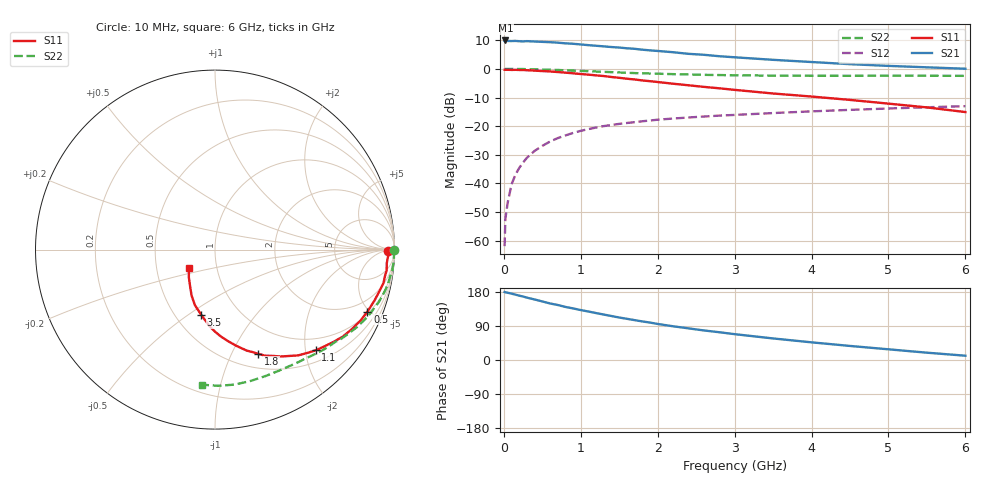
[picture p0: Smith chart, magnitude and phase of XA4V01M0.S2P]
! SIEMENS Discrete & RF Semiconductors
! BFY180
! Si NPN RF Bipolar Junction Transistor in MICRO-X
! VCE = 4 V  IC = 1 mA
! Common Emitter S-Parameters:  May  1997
# GHz  S  MA  R  50
!  f  S11  S21  S12  S22
! GHz  MAG  ANG  MAG  ANG  MAG  ANG  MAG  ANG
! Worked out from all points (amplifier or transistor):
!   36 points, 10 MHz to 6 GHz, reference 50 ohm
!   highest |S21| = 9.9 dB at 20 MHz (marker M1)
!   |S21| within 3 dB of that: start of sweep to 1.726 GHz
!   unconditionally stable (mu >= 1): 3.982 GHz to end of sweep
!   at 250 MHz: K = 0.06, MSG = 21.2 dB, |S12| = -32.7 dB
!   at 1.4 GHz: K = 0.50, MSG = 13.6 dB, |S12| = -19.6 dB
!   at 6 GHz: K = 1.06, MAG = 5.1 dB, |S12| = -13.0 dB
!   S11 on the Smith chart (normalised r, x): 10 MHz: 56, -8; 500 MHz: 1.12, -4.87; 1.1 GHz: 0.73, -2.21; 1.8 GHz: 0.66, -1.27; 3.5 GHz: 0.67, -0.56; 6 GHz: 0.73, -0.15
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0.01  0.9657 -0.3  3.059 179.4  0.0008 73.3  0.9984 -0.2
0.02  0.9643 -0.9  3.141 178.6  0.0024 84.6  0.9999 -0.5
0.05  0.9654 -2.0  3.077 177.5  0.0046 84.1  0.9968 -1.3
0.1  0.96 -4.5  3.065 175.1  0.0096 87.6  0.9979 -2.7
0.15  0.9634 -6.9  3.084 172.5  0.0141 85.5  0.9983 -4.0
0.25  0.957 -11.2  3.025 167.5  0.0232 83.5  0.9947 -6.7
0.3  0.9483 -13.3  3.056 164.6  0.028 81.0  0.9888 -7.9
0.5  0.9169 -22.1  2.968 154.5  0.0452 74.6  0.9767 -13.0
0.6  0.9022 -26.0  2.929 149.2  0.0538 71.7  0.9674 -15.5
0.7  0.8817 -30.2  2.876 145.2  0.0617 68.7  0.9578 -17.9
0.8  0.861 -34.3  2.797 140.1  0.0688 66.4  0.9451 -20.2
1.1  0.7938 -45.0  2.6 127.9  0.0888 58.8  0.9118 -26.6
1.5  0.6993 -58.4  2.361 112.1  0.1096 50.6  0.8672 -34.2
1.8  0.6292 -67.4  2.167 101.8  0.1217 45.9  0.8378 -39.1
2.2  0.5513 -77.2  1.956 89.0  0.1358 40.2  0.8104 -45.3
2.6  0.4855 -86.1  1.765 78.0  0.1472 36.0  0.7876 -50.6
3  0.4303 -93.8  1.596 68.2  0.1571 31.9  0.7737 -55.9
3.5  0.3718 -101.9  1.441 56.9  0.1693 28.0  0.7631 -62.0
4  0.3291 -109.9  1.319 46.6  0.1812 23.9  0.7587 -68.4
4.5  0.2873 -117.0  1.21 37.1  0.1925 20.1  0.7582 -75.0
5.5  0.2124 -133.3  1.066 19.3  0.2138 12.4  0.7591 -88.7
6  0.1763 -145.3  1.007 11.3  0.2235 8.2  0.7563 -95.6
